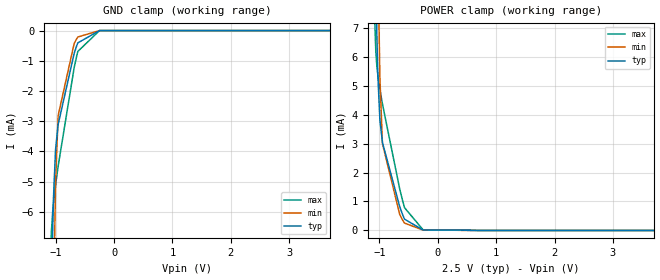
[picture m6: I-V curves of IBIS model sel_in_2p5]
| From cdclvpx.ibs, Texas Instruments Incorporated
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|   Sel_in_2p5 Model   |
[Model]   sel_in_2p5
Model_type   Input
Vinl = 0.11
Vinh = 1.36
|   typ   min   max
|   (nom PVT)   (fast PVT)   (slow PVT)
C_comp   1.868e-13   1.723e-13   2.073e-13
| Where nom  PVT is Nominal Process, 2.5V, 40C
|   Fast PVT is Strong Process,  2.625V, -40C
|   Slow PVT is Weak Process,   2.375V,100C
[Voltage Range]   2.5   2.375   2.625
|Junction Temperature
[Power Clamp Reference]   2.5   2.375   2.625
[GND Clamp Reference]   0   0   0
[GND Clamp]
|   Voltage   I(typ)   I(min)   I(max)
-2.5V     -665.9mA   -674.2mA   -658.7mA
-1.073V   -9.032mA   -15.7mA    -6.624mA
-1.051V   -6.564mA   -11.31mA   -5.991mA
-1.038V   -5.54mA    -9.143mA   -5.716mA
-1.004V   -4.002mA   -5.227mA   -5.148mA
-999mV    -3.87mA    -4.855mA   -5.077mA
-958.6mV  -3.119mA   -2.847mA   -4.5mA
-957.5mV  -3.103mA   -2.813mA   -4.485mA
-683.1mV  -750.8uA   -425.2uA   -1.221mA
-620.5mV  -407.4uA   -212.5uA   -690.8uA
-250mV    -50.26nA   -68.38nA   0A
5V        0A         0A         0A
[POWER Clamp]
|   Voltage   I(typ)   I(min)   I(max)
-2.5V     671.4mA    680mA      664.2mA
-1.093V   14.45mA    23.87mA    7.99mA
-1.063V   9.023mA    16.22mA    6.207mA
-1.046V   6.879mA    12.51mA    5.703mA
-1.027V   5.348mA    9.33mA     5.351mA
-992.5mV  3.823mA    5.305mA    4.873mA
-948.6mV  3.036mA    2.993mA    4.365mA
-652.2mV  817.6uA    549.3uA    1.426mA
-570.6mV  391.1uA    255.3uA    787.5uA
-250mV    13.21uA    10.44uA    17.49uA
5V        0A         0A         0A
